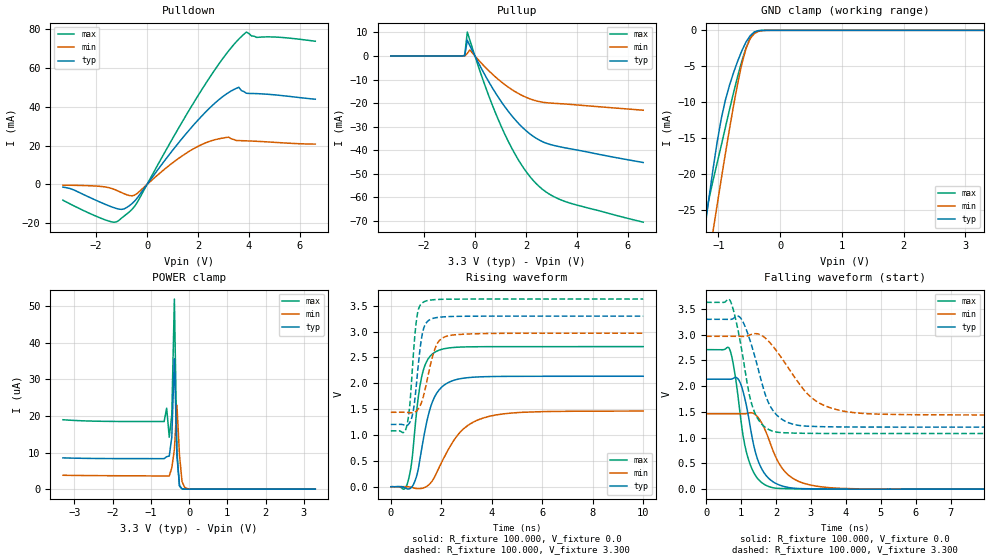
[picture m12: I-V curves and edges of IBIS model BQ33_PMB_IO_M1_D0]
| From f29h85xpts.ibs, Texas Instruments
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|   Model BQ33_PMB_IO_M1_D0
[Model]   BQ33_PMB_IO_M1_D0
Model_type   I/O
Polarity   Non-Inverting
Enable   Active-Low
Vinl =   0.800V
Vinh =   1.350V
Vmeas =  1.650V
Cref =   10.000pF
Vref =   0.0V
|   typ   min   max
C_comp   1.786pF   1.720pF   1.856pF
[Model Spec]
Vinh   1.350V   1.350V   1.350V
Vinl   0.800V   0.800V   0.800V
[Temperature Range]   30   155   -40
[Voltage Range]   3.300V   2.970V   3.630V
[Pullup Reference]   3.300V   2.970V   3.630V
[Pulldown Reference]   0.0V   0.0V   0.0V
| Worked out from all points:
|   slope of the pulldown table from 0 to 0.495 V, typ, clamps not added: 55.8 ohm
|   slope of the pullup table from 0 to 0.495 V, typ, clamps not added: 49.3 ohm
|   GND clamp passes 1 mA (typ) near -0.51 V on its own axis
|   rising waveform, R_fixture 100.000, V_fixture 0.0: 20-80 % time 589ps typ, 1.18ns min, 398ps max; typ from 0 V to 2.14 V
|   rising waveform, R_fixture 100.000, V_fixture 3.300: 20-80 % time 286ps typ, 456ps min, 238ps max; typ from 1.21 V to 3.3 V
|   falling waveform, R_fixture 100.000, V_fixture 0.0: 20-80 % time 441ps typ, 650ps min, 389ps max; typ from 2.14 V to 0 V
|   falling waveform, R_fixture 100.000, V_fixture 3.300: 20-80 % time 565ps typ, 1.03ns min, 430ps max; typ from 3.3 V to 1.21 V
[Pulldown]
|Voltage   I(typ)   I(min)   I(max)
-3.3V     -1.377mA   -345.3uA   -8.105mA
-1.6V     -10.44mA   -1.376mA   -18.44mA
-1.1V     -12.71mA   -3.587mA   -18.49mA
-500mV    -8.748mA   -5.575mA   -11.5mA
1.3V      22.5mA     14.03mA    30.49mA
2.5V      39.99mA    22.45mA    56.04mA
3.2V      47.44mA    24.4mA     68.91mA
3.5V      49.58mA    22.7mA     73.6mA
3.8V      47.94mA    22.56mA    77.52mA
3.9V      47.06mA    22.51mA    78.61mA
4.3V      46.87mA    22.28mA    75.86mA
6.6V      43.99mA    20.83mA    73.9mA
[Pullup]
|Voltage   I(typ)   I(min)   I(max)
-3.3V     194.8pA    12.42nA    5.76nA
-500mV    17.31nA    18.01nA    59.06nA
-400mV    178uA      374.8nA    408.1uA
-300mV    6.695mA    1.073mA    10.14mA
-200mV    4.421mA    2.585mA    6.742mA
400mV     -8.225mA   -4.706mA   -12.71mA
1V        -18.86mA   -10.69mA   -29.11mA
1.7V      -28.5mA    -15.89mA   -44mA
2.3V      -34.18mA   -18.71mA   -52.97mA
2.8V      -37.02mA   -19.82mA   -57.77mA
3.5V      -38.88mA   -20.34mA   -61.58mA
6.6V      -45.18mA   -23.01mA   -70.51mA
[GND_clamp]
|Voltage   I(typ)   I(min)   I(max)
-3.3V     -172.4mA   -156.6mA   -199.3mA
-1.223V   -27.66mA   -35.43mA   -26.88mA
-1.156V   -23.42mA   -31.69mA   -23.54mA
-1.089V   -19.35mA   -27.98mA   -20.9mA
-1.022V   -15.58mA   -24.31mA   -18.47mA
-955mV    -12.3mA    -20.69mA   -16.02mA
-821mV    -7.634mA   -13.71mA   -11.02mA
-620mV    -2.823mA   -4.633mA   -4.248mA
-553mV    -1.627mA   -2.509mA   -2.447mA
-419mV    -233.8uA   -453.9uA   -289uA
-218mV    -985nA     -9.253uA   -449.5nA
3.3V      0A         0A         0A
[POWER_clamp]
|Voltage   I(typ)   I(min)   I(max)
-3.3V     8.55uA     3.797uA    18.96uA
-653mV    8.339uA    3.596uA    18.47uA
-586mV    8.872uA    3.591uA    22.11uA
-519mV    9.031uA    3.588uA    14.17uA
-452mV    14.26uA    5.833uA    20.33uA
-385mV    35.62uA    10.82uA    51.91uA
-318mV    9.151uA    22.94uA    10.03uA
-251mV    942nA      9.217uA    856.3nA
-184mV    84.85nA    2.059uA    62.73nA
-117mV    8.015nA    524.6nA    4.599nA
-50mV     1.476nA    168.6nA    663.4pA
3.3V      0A         0A         0A
[Ramp]
| variable   typ   min   max
dV/dt_r   1.282/0.589n   0.878/1.175n   1.626/0.398n
dV/dt_f   1.257/0.565n   0.917/1.035n   1.530/0.430n
R_load = 100.000
[Rising Waveform]
R_fixture= 100.000
V_fixture= 0.0
V_fixture_min= 0.0
V_fixture_max= 0.0
|time   V(typ)   V(min)   V(max)
0s        15.49uV    21.03uV    14.63uV
643ps     -40.91mV   1.751mV    41.74mV
816ps     -14.4mV    -10.84mV   432.8mV
966ps     123.4mV    -30.47mV   1.176V
1.218ns   718.9mV    -31.89mV   2.115V
1.498ns   1.407V     34.86mV    2.486V
1.787ns   1.784V     242.3mV    2.614V
2.665ns   2.081V     1.009V     2.699V
3.655ns   2.128V     1.329V     2.709V
10ns      2.137V     1.464V     2.71V
[Rising Waveform]
R_fixture= 100.000
V_fixture= 3.300
V_fixture_min= 2.970
V_fixture_max= 3.630
|time   V(typ)   V(min)   V(max)
0s        1.205V     1.441V     1.08V
631ps     1.185V     1.44V      1.173V
741ps     1.234V     1.434V     1.526V
859ps     1.395V     1.432V     2.31V
1.028ns   2.051V     1.47V      3.264V
1.17ns    2.711V     1.575V     3.515V
1.308ns   3.071V     1.781V     3.575V
1.754ns   3.266V     2.675V     3.619V
2.192ns   3.289V     2.908V     3.627V
10ns      3.3V       2.97V      3.63V
[Falling Waveform]
R_fixture= 100.000
V_fixture= 0.0
V_fixture_min= 0.0
V_fixture_max= 0.0
|time   V(typ)   V(min)   V(max)
0s        2.137V     1.465V     2.71V
676ps     2.136V     1.465V     2.715V
791ps     2.158V     1.465V     2.377V
943ps     2.113V     1.464V     1.638V
1.179ns   1.535V     1.472V     653.7mV
1.44ns    649.3mV    1.428V     237.6mV
1.775ns   220.9mV    1.005V     56.14mV
2.29ns    41.92mV    315.4mV    9.798mV
3.096ns   6.204mV    65.38mV    2.027mV
10ns      13.29uV    53.99uV    28.12uV
[Falling Waveform]
R_fixture= 100.000
V_fixture= 3.300
V_fixture_min= 2.970
V_fixture_max= 3.630
|time   V(typ)   V(min)   V(max)
0s        3.3V       2.97V      3.63V
691ps     3.298V     2.97V      3.659V
998ps     3.315V     2.969V     2.784V
1.326ns   2.737V     3.014V     1.607V
1.553ns   2.172V     2.999V     1.295V
1.863ns   1.579V     2.817V     1.137V
2.253ns   1.323V     2.456V     1.096V
2.902ns   1.224V     1.85V      1.085V
3.772ns   1.209V     1.538V     1.082V
10ns      1.205V     1.442V     1.08V
